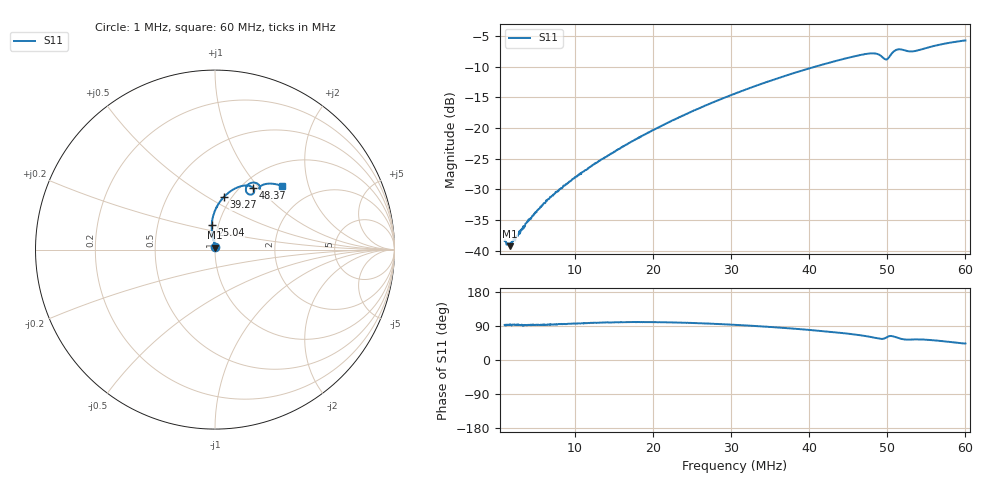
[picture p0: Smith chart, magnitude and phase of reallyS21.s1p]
! ListType=Lin
!!2 x 2 x FT290-43 mit 2 x 2 x 6 Windungen mit AWG12 mit Ueberschlag
# MHz S RI R 50
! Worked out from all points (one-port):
!   1000 points, 1 MHz to 60 MHz, reference 50 ohm
!   lowest |S11| = -39.3 dB at 1.65 MHz (marker M1), VSWR 1.02, Z = 49.9 + j1.08 ohm
!   |S11| at or under -10 dB: start of sweep to 40.83 MHz
!   S11 on the Smith chart (normalised r, x): 1 MHz: 1.00, +0.02; 25.04 MHz: 0.93, +0.26; 39.27 MHz: 0.92, +0.59; 48.37 MHz: 1.12, +0.93; 60 MHz: 1.41, +1.37
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1  -0.000513 0.012
1.64965  -0.000738 0.0109
2.417417  -0.000527 0.0127
3.952953  -0.000612 0.0172
5.075075  -0.00103 0.0205
6.610611  -0.0013 0.0263
8.382382  -0.00272 0.0325
12.22122  -0.00711 0.0492
15.76476  -0.0113 0.0669
23.14715  -0.0182 0.1189
25.03704  -0.018 0.1358
30.52953  -0.00926 0.1908
37.91191  0.0351 0.2759
39.27027  0.0481 0.2919
45.29429  0.1368 0.3508
47.12513  0.1781 0.3572
48.36537  0.2095 0.3459
49.07407  0.2187 0.3239
49.60561  0.201 0.306
49.95996  0.1789 0.3149
50.31431  0.1727 0.3424
50.78679  0.1951 0.3691
51.25926  0.2239 0.372
51.90891  0.248 0.3563
52.67668  0.2501 0.3397
54.56657  0.2578 0.3562
56.86987  0.3071 0.3675
60  0.3727 0.3562
